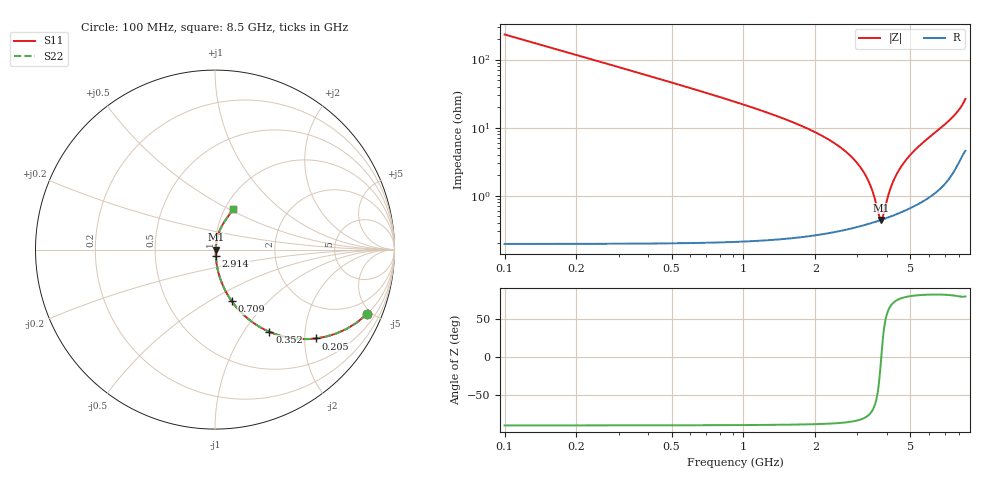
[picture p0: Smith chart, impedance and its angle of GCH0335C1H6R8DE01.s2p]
!Murata Part Number: GCH0335C1H6R8DE01
!These Parameters are Measured in Series Mode Connection
!Data Generated on Mar 13, 2026
!  o--ll--o
!Port1  Port2
!  o------o
!Operation Temp=25[degC], DC Bias Voltage=0[V]
!Freq. Start=100[MHz] Stop=9[GHz] 401[Steps]
# Hz S RI R 50
!Freq.(Hz) S11(Real) S11(Imag) S21(Real) S21(Imag) S12(Real) S12(Imag) S22(Real) S22(Imag)
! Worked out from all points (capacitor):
!   401 points, 100 MHz to 8.5 GHz, reference 50 ohm
!   read as one part in series: C = 6.8 pF near 142 MHz
!   lowest |Z| = 440 mohm at 3.775 GHz (marker M1)
!   series resonance near 3.776 GHz, so ESL is about 260 pH
!   S11 on the Smith chart (normalised r, x): 100 MHz: 1.00, -4.68; 205 MHz: 1.00, -2.28; 352 MHz: 1.00, -1.32; 709 MHz: 1.00, -0.64; 2.914 GHz: 1.01, -0.07; 8.5 GHz: 1.09, +0.52
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1e8  0.8452 -0.3613  0.1548 0.3613  0.1548 0.3613  0.8452 -0.3613
2.05e8  0.5644 -0.495  0.4356 0.495  0.4356 0.495  0.5644 -0.495
3.52e8  0.3036 -0.4583  0.6964 0.4583  0.6964 0.4583  0.3036 -0.4583
4.99e8  0.1765 -0.3791  0.8235 0.3791  0.8235 0.3791  0.1765 -0.3791
7.09e8  0.0939 -0.2885  0.9061 0.2885  0.9061 0.2885  0.0939 -0.2885
1.507e9  0.0192 -0.1287  0.9808 0.1287  0.9808 0.1287  0.0192 -0.1287
2.41e9  0.00631 -0.0582  0.9937 0.0582  0.9937 0.0582  0.00631 -0.0582
2.914e9  0.00447 -0.0332  0.9955 0.0332  0.9955 0.0332  0.00447 -0.0332
3.166e9  0.00414 -0.0226  0.9959 0.0226  0.9959 0.0226  0.00414 -0.0226
3.355e9  0.00407 -0.0152  0.9959 0.0152  0.9959 0.0152  0.00407 -0.0152
3.502e9  0.00412 -0.00971  0.9959 0.00971  0.9959 0.00971  0.00412 -0.00971
3.712e9  0.0043 -0.00222  0.9957 0.00222  0.9957 0.00222  0.0043 -0.00222
3.775e9  0.00438 -4.53e-05  0.9956 4.53e-05  0.9956 4.53e-05  0.00438 -4.53e-05
3.838e9  0.00447 0.0021  0.9955 -0.0021  0.9955 -0.0021  0.00447 0.0021
4.09e9  0.00495 0.0105  0.995 -0.0105  0.995 -0.0105  0.00495 0.0105
4.3e9  0.00547 0.0172  0.9945 -0.0172  0.9945 -0.0172  0.00547 0.0172
4.552e9  0.00625 0.0251  0.9938 -0.0251  0.9938 -0.0251  0.00625 0.0251
4.846e9  0.00735 0.034  0.9926 -0.034  0.9926 -0.034  0.00735 0.034
5.707e9  0.012 0.0604  0.988 -0.0604  0.988 -0.0604  0.012 0.0604
7.114e9  0.0289 0.1124  0.9711 -0.1124  0.9711 -0.1124  0.0289 0.1124
7.975e9  0.0579 0.1636  0.9421 -0.1636  0.9421 -0.1636  0.0579 0.1636
8.5e9  0.0997 0.2248  0.9003 -0.2248  0.9003 -0.2248  0.0997 0.2248
